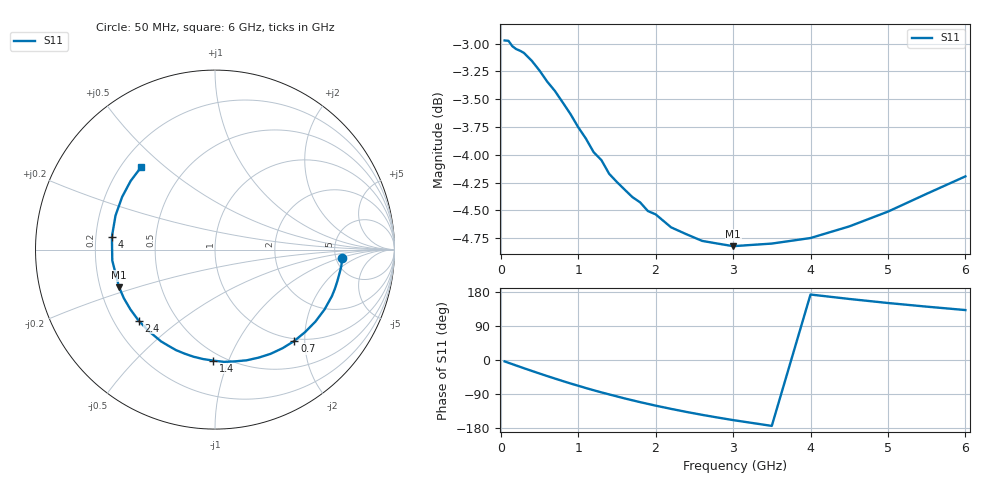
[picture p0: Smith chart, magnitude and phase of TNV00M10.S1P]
! SIEMENS Discrete & RF Semiconductors
! BAS70-07W
! Si Schottky Diode in SOT343
! IF = 0.1 mA
! S-Parameters:  February  1997
# GHz  S  MA  R  50
!  f  S11
! GHz  MAG  ANG
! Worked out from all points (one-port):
!   34 points, 50 MHz to 6 GHz, reference 50 ohm
!   lowest |S11| = -4.8 dB at 3 GHz (marker M1), VSWR 3.70, Z = 14 - j8.73 ohm
!   |S11| at or under -10 dB: nowhere
!   S11 on the Smith chart (normalised r, x): 50 MHz: 5.70, -1.05; 700 MHz: 0.96, -1.79; 1.4 GHz: 0.44, -0.88; 2.4 GHz: 0.30, -0.36; 4 GHz: 0.27, +0.06; 6 GHz: 0.28, +0.42
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0.05  0.7102 -3.7
0.1  0.7099 -7.4
0.15  0.706 -10.9
0.3  0.7011 -21.7
0.4  0.6955 -28.7
0.5  0.6885 -35.6
0.6  0.6806 -42.4
0.7  0.674 -49.0
0.8  0.6661 -55.5
0.9  0.6582 -61.9
1  0.6493 -67.9
1.1  0.6416 -74.0
1.3  0.6275 -85.4
1.4  0.6187 -90.8
1.6  0.6086 -101.4
1.8  0.6007 -111.2
2  0.5933 -120.4
2.2  0.5853 -129.0
2.4  0.5811 -137.1
2.6  0.5772 -144.7
2.8  0.5756 -151.8
3  0.574 -158.6
3.5  0.5756 -173.9
4  0.5789 172.8
4.5  0.5859 161.1
5  0.5949 150.4
5.5  0.606 140.8
6  0.617 131.8
